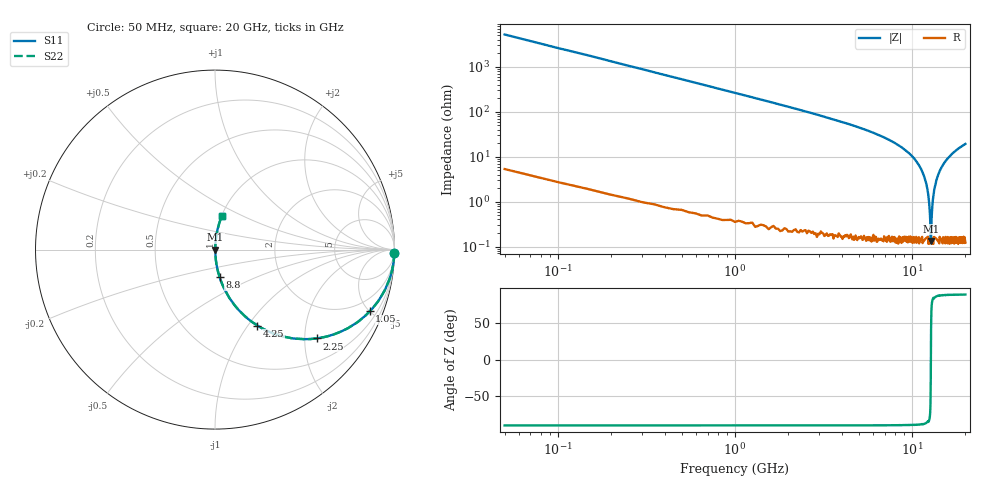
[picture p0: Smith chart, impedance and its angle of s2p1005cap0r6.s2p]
!	AVX	Thin	Film	Operation
!	Date:	March 2012
!	Description: Ultra-Miniature 01005 Size ACCU - P® Thin Film RF / Microwave Capacitor
!	Part Number:  C005YJ0R6ABSTR
!	Serial	Measurements
# MHZ S MA R 50
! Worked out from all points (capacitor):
!   400 points, 50 MHz to 20 GHz, reference 50 ohm
!   read as one part in series: C = 598 fF near 150 MHz
!   lowest |Z| = 132 mohm at 12.75 GHz (marker M1)
!   series resonance near 12.77 GHz, so ESL is about 260 pH
!   S11 on the Smith chart (normalised r, x): 50 MHz: open; 1.05 GHz: 1.01, -5.02; 2.25 GHz: 1.00, -2.29; 4.25 GHz: 1.00, -1.11; 8.8 GHz: 1.00, -0.32; 20 GHz: 1.00, +0.39
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50  1 -1.1  0.019 88.9  0.019 88.9  1 -1.1
150  0.998 -3.2  0.056 86.7  0.056 86.7  0.998 -3.2
350  0.991 -7.5  0.131 82.4  0.131 82.4  0.991 -7.5
1050  0.928 -21.7  0.37 68.2  0.37 68.2  0.928 -21.7
2250  0.752 -41.2  0.658 48.7  0.658 48.7  0.752 -41.2
3400  0.586 -54.0  0.809 35.9  0.809 35.9  0.586 -54.0
4250  0.485 -60.8  0.873 29.0  0.873 29.0  0.485 -60.8
6700  0.275 -73.7  0.96 16.0  0.96 16.0  0.275 -73.7
8800  0.156 -80.5  0.986 9.0  0.986 9.0  0.156 -80.5
10050  0.1 -83.5  0.994 5.7  0.994 5.7  0.1 -83.5
11250  0.053 -85.5  0.997 3.0  0.997 3.0  0.053 -85.5
12150  0.021 -84.9  0.998 1.2  0.998 1.2  0.021 -84.9
12550  0.007254 -78.5  0.999 0.4  0.999 0.4  0.007254 -78.5
12650  0.004072 -69.8  0.999 0.2  0.999 0.2  0.004072 -69.8
12750  0.001501 -21.8  0.999 0.0  0.999 0.0  0.001501 -21.8
12800  0.001754 37.3  0.999 -0.1  0.999 -0.1  0.001754 37.3
12900  0.004515 71.8  0.999 -0.2  0.999 -0.2  0.004515 71.8
13000  0.007628 79.0  0.999 -0.4  0.999 -0.4  0.007628 79.0
13350  0.019 84.6  0.998 -1.1  0.998 -1.1  0.019 84.6
14600  0.056 85.4  0.997 -3.2  0.997 -3.2  0.056 85.4
16700  0.112 82.8  0.992 -6.4  0.992 -6.4  0.112 82.8
20000  0.189 78.7  0.981 -10.9  0.981 -10.9  0.189 78.7
